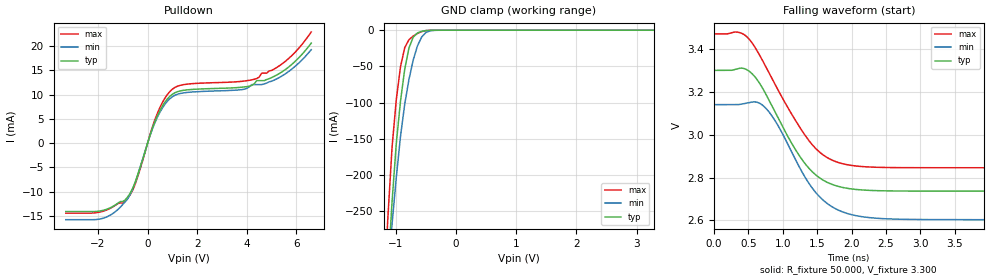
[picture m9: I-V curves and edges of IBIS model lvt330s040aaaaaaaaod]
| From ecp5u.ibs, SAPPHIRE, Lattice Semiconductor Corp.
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|   Model lvt330s040aaaaaaaaod
[Model] lvt330s040aaaaaaaaod
Model_type I/O_open_drain
Polarity   Non-Inverting
Enable   Active-Low
Vinl =  0.800V
Vinh =  2.000V
Vmeas =  1.650V
Cref =  0.0F
Rref =  1.000M
Vref =  3.3V
C_comp   5.000pF   4.000pF   5.500pF
[Temperature Range]   25.000   0.125k   -40.000
[Voltage Range]   3.300V   3.140V   3.470V
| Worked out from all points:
|   slope of the pulldown table from 0 to 0.495 V, typ, clamps not added: 73.9 ohm
|   GND clamp passes 1 mA (typ) near -0.54 V on its own axis
|   falling waveform, R_fixture 50.000, V_fixture 3.300: 20-80 % time 606ps typ, 585ps min, 676ps max; typ from 3.3 V to 2.74 V
[Pulldown]
|Voltage   I(typ)   I(min)   I(max)
-3.3V     -14.12mA   -15.79mA   -14.44mA
-1.8V     -13.87mA   -15.5mA    -14.05mA
-800mV    -11.08mA   -11.47mA   -11.33mA
-500mV    -8.065mA   -8.084mA   -8.464mA
300mV     4.505mA    4.281mA    4.905mA
600mV     7.672mA    7.282mA    8.406mA
1V        10.09mA    9.572mA    11.13mA
1.6V      10.99mA    10.46mA    12.17mA
4V        11.65mA    11.3mA     12.87mA
4.4V      12.89mA    12.07mA    13.33mA
5.5V      14.97mA    14.11mA    16.65mA
6.6V      20.62mA    19.27mA    22.93mA
[GND_clamp]
|Voltage   I(typ)   I(min)   I(max)
-3.3V     -4.927A    -3.455A    -6.917A
-1.2V     -438mA     -409mA     -376.6mA
-1.13V    -332.7mA   -335.8mA   -258.9mA
-1.06V    -236.4mA   -267mA     -161mA
-990mV    -156.1mA   -203.1mA   -95.6mA
-920mV    -97.57mA   -146.3mA   -50.22mA
-850mV    -53.64mA   -101.9mA   -23.95mA
-780mV    -24.57mA   -67.95mA   -13.06mA
-640mV    -3.835mA   -21.83mA   -4.519mA
-500mV    -471.8uA   -3.197mA   -537.5uA
-360mV    -15.56uA   -174.4uA   -12.69uA
3.28V     0A         0A         0A
[Ramp]
| variable   typ   min   max
dV/dt_r   0.338/1.202n   0.322/1.651n   0.375/0.445n
dV/dt_f   0.338/0.612n   0.322/0.595n   0.375/0.683n
R_load = 50.000
[Falling Waveform]
R_fixture= 50.000
V_fixture= 3.300
V_fixture_min= 3.140
V_fixture_max= 3.470
|time   V(typ)   V(min)   V(max)
0s        3.3V       3.14V      3.47V
429ps     3.31V      3.144V     3.469V
569ps     3.28V      3.153V     3.422V
716ps     3.213V     3.135V     3.341V
923ps     3.084V     3.047V     3.214V
1.353ns   2.853V     2.786V     2.984V
1.609ns   2.784V     2.688V     2.901V
1.933ns   2.75V      2.632V     2.86V
2.953ns   2.737V     2.604V     2.846V
10ns      2.736V     2.603V     2.846V
